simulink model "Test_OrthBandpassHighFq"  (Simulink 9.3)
settings: Solver=VariableStepAuto  StartTime=0.0  StopTime=10  RelTol=1e-3
InitFcn:
  | Test_LibVishia_Ctrl.TestOrthOsc_init()
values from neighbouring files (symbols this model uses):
  Tstep = 0.000050    (= 5e-05)    [TestOrthOsc_init.m]    (also in Test_PIDctrl_init.m = 0.0001)
libraries: libVishia_Ctrl x3, libVishia_Conv x2

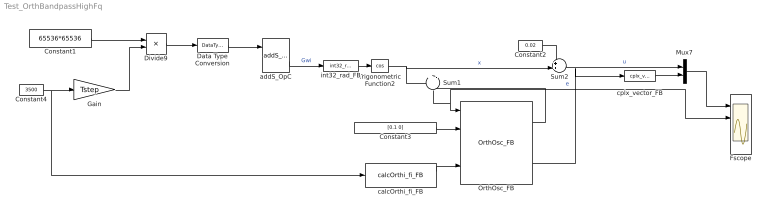
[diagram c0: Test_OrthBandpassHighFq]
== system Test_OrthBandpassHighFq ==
  Constant1 : Constant  Value=65536*65536  OutDataTypeStr=single
  Constant2 : Constant  Value=0.02  OutDataTypeStr=single
  Constant3 : Constant  Value=[0.1 0]  OutDataTypeStr=single
  Constant4 : Constant  Value=3500  OutDataTypeStr=single
  Data Type Conversion : DataTypeConversion  OutDataTypeStr=int32
  Divide9 : Product  Inputs=**
  Fscope : Scope  NumInputPorts=4
  Gain : Gain  Gain=Tstep
  Mux7 : Mux  Inputs=2
  OrthOsc_FB : libVishia_Ctrl/OrthOsc_FB
  Sum1 : Sum  Inputs=+|-
  Sum2 : Sum  Inputs=++|
  Trigonometric Function2 : Trigonometry  Operator=cos
  addS_OpC : libVishia_Ctrl/addS_OpC  init=0  Tstep=Tstep
  calcOrthi_fi_FB : libVishia_Ctrl/calcOrthi_fi_FB  Tstep=Tstep
  cplx_vector_FB : libVishia_Conv/cplx_vector_FB  SystemSampleTime=-1
  int32_rad_FB : libVishia_Conv/int32_rad_FB  SystemSampleTime=-1
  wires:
  ? -> ?
  Constant3/1 -> OrthOsc_FB/3
  calcOrthi_fi_FB/1 -> OrthOsc_FB/7
  Constant4/1 -> calcOrthi_fi_FB/1, Gain/1
  Data Type Conversion/1 -> addS_OpC/1
  int32_rad_FB/1 -> Trigonometric Function2/1
  addS_OpC/2 -> int32_rad_FB/1  "Gwi"
  Divide9/1 -> Data Type Conversion/1
  Gain/1 -> Divide9/2
  Trigonometric Function2/1 -> Sum2/2, Sum1/1  "x"
  Constant1/1 -> Divide9/1
  Mux7/1 -> Fscope/1
  cplx_vector_FB/1 -> Mux7/2
  OrthOsc_FB/3 -> cplx_vector_FB/1
  OrthOsc_FB/1 -> Sum1/2
  Sum1/1 -> Fscope/2, OrthOsc_FB/1  "e"
  Sum2/1 -> Mux7/1  "u"
  Constant2/1 -> Sum2/1
